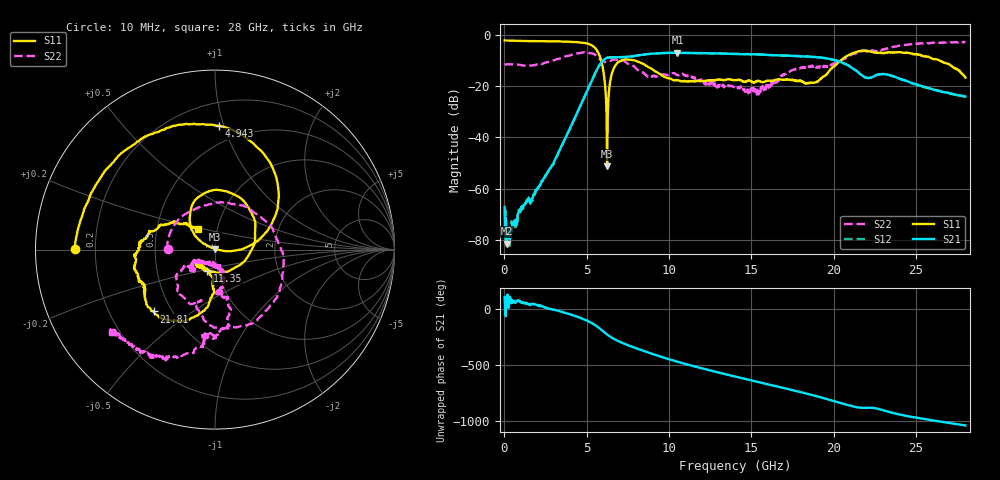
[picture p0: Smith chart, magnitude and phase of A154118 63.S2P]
!  2-Port S-parameters saved by WinCal
! VAR MeasName=S-Parameters (CALIBRATED_DATA) read from VNA (N5230A)
! VAR MeasDate=2015-9-10 14:40:00
! VAR NAME=A154118 63
! VAR FILENAME=A154118 63.S2P
! VAR DATE=2015-9-10 14:40:00
! VAR PHYS_PORTS=1,2
# Hz S DB R 50
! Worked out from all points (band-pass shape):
!   801 points, 10 MHz to 28 GHz, reference 50 ohm
!   highest |S21| = -6.96 dB at 10.51 GHz (marker M1); lowest = -81.5 dB at 149.9 MHz (marker M2)
!   |S21| within 3 dB of the highest: 5.993 GHz to 20.15 GHz (14.16 GHz wide, 108 % of centre)
!   lowest |S11| = -51.2 dB at 6.238 GHz (marker M3), VSWR 1.01, Z = 50.2 + j0.21 ohm
!   |S11| at or under -10 dB: 5.875 GHz to 7.102 GHz (1.227 GHz wide, 18.9 % of centre); 7.943 GHz to 20.42 GHz (12.48 GHz wide, 88 % of centre); 26.42 GHz to end of sweep
!   |S22| runs from -23.3 to -2.7 dB; largest |S21 - S12| = 0.0083
!   S11 on the Smith chart (normalised r, x): 10 MHz: 0.12, +0.00; 4.943 GHz: 0.36, +0.96; 11.35 GHz: 0.89, -0.21; 21.81 GHz: 0.40, -0.36; 28 GHz: 0.81, +0.19
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1e7  -2.15 179.7  -67.21 105.3  -74.56 -174.7  -11.64 179.7
1.4995e8  -2.16 177.7  -81.47 63.0  -82.51 99.1  -11.45 172.6
2.564088e9  -2.46 145.3  -54.51 11.1  -54.45 12.5  -10.70 55.5
3.753662e9  -2.60 123.8  -39.59 -35.6  -39.63 -35.9  -8.24 -6.6
4.698325e9  -3.04 98.2  -26.50 -82.5  -26.49 -83.0  -6.92 -55.7
4.943238e9  -3.22 88.3  -22.96 -97.2  -23.01 -96.9  -6.80 -67.3
5.782938e9  -8.16 29.9  -11.69 -172.2  -11.68 -172.3  -9.38 -107.6
6.237775e9  -51.23 49.7  -8.96 133.5  -8.94 133.5  -10.68 -105.3
6.552662e9  -14.58 136.7  -8.72 102.5  -8.71 102.2  -9.78 -111.9
6.972512e9  -10.41 109.6  -8.69 70.2  -8.67 69.9  -9.99 -124.9
8.197075e9  -10.71 47.5  -7.89 -0.0  -7.88 -0.0  -14.20 -151.1
9.351662e9  -14.89 -18.3  -7.18 -58.1  -7.13 -58.1  -16.30 -137.0
1.050625e10  -17.65 -82.8  -6.96 -109.9  -6.96 -110.4  -15.73 -141.1
1.134595e10  -18.00 -110.0  -7.08 -144.2  -7.05 -144.6  -16.24 -148.3
1.4005e10  -17.67 -144.1  -7.43 117.7  -7.41 117.2  -20.38 -131.4
1.662906e10  -17.36 -137.0  -7.95 26.5  -7.92 25.7  -17.32 -69.7
1.869332e10  -18.56 -117.4  -8.56 -47.8  -8.60 -48.3  -11.93 -85.6
2.051268e10  -9.59 -98.8  -10.83 -123.4  -10.81 -124.2  -9.62 -76.1
2.180721e10  -6.29 -134.7  -16.12 -162.5  -16.21 -163.1  -6.09 -89.7
2.334666e10  -6.84 -157.2  -15.61 161.3  -15.63 160.1  -5.24 -98.8
2.628561e10  -9.56 155.1  -21.67 78.9  -21.69 78.0  -3.03 -128.3
2.8e10  -16.63 129.0  -24.03 40.0  -24.10 39.6  -2.71 -141.3
